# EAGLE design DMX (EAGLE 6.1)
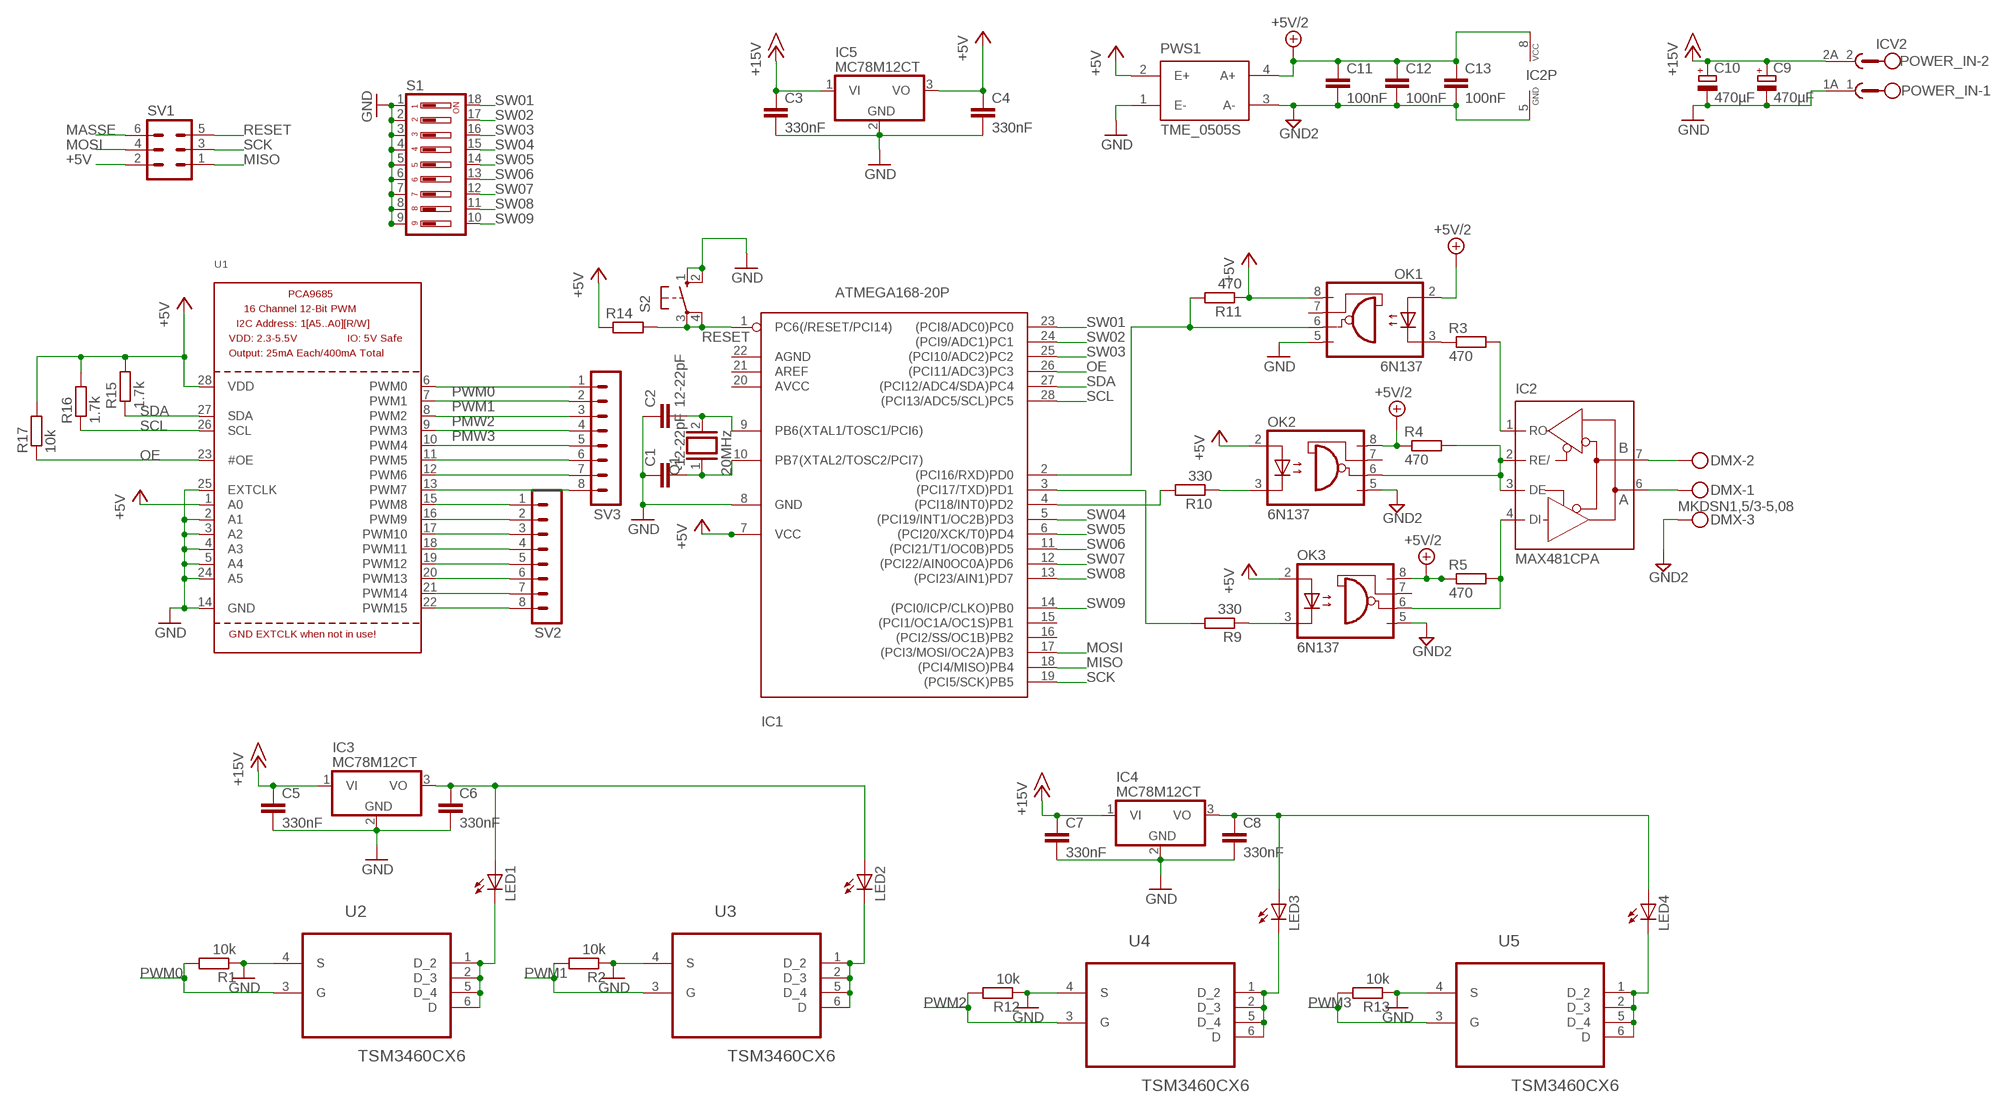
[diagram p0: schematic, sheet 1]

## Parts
C1  12-22pF  C-EU025-025X050  [C025-025X050]
C2  12-22pF  C-EU025-025X050  [C025-025X050]
C3  330nF  C-EU050-025X075  [C050-025X075]
C4  330nF  C-EU050-025X075  [C050-025X075]
C5  330nF  C-EU050-025X075  [C050-025X075]
C6  330nF  C-EU050-025X075  [C050-025X075]
C7  330nF  C-EU050-025X075  [C050-025X075]
C8  330nF  C-EU050-025X075  [C050-025X075]
C9  470µF  CPOL-EUE5-10.5  [E5-10,5]
C10  470µF  CPOL-EUE5-10.5  [E5-10,5]
C11  100nF  C-EU050-025X075  [C050-025X075]
C12  100nF  C-EU050-025X075  [C050-025X075]
C13  100nF  C-EU050-025X075  [C050-025X075]
DMX  MKDSN1,5/3-5,08  [MKDSN1,5/3-5,08]
IC1  ATMEGA168-20P  [DIL28-3]
IC2  MAX481CPA  [DIL08]
IC3  MC78M12CT  [TO220V]
IC4  MC78M12CT  [TO220V]
IC5  MC78M12CT  [TO220V]
LED1  LED5MM  [LED5MM]
LED2  LED5MM  [LED5MM]
LED3  LED5MM  [LED5MM]
LED4  LED5MM  [LED5MM]
OK1  6N137  [DIL08]
OK2  6N137  [DIL08]
OK3  6N137  [DIL08]
POWER_IN  ICV2  [ICV2]
PWS1  TME_0505S  [TMEXXXXS]
Q1  20MHz  XTAL/S  [QS]
R1  10k  R-EU_0207/7  [0207/7]
R2  10k  R-EU_0207/7  [0207/7]
R3  470  R-EU_0207/7  [0207/7]
R4  470  R-EU_0207/7  [0207/7]
R5  470  R-EU_0207/7  [0207/7]
R9  330  R-EU_0207/7  [0207/7]
R10  330  R-EU_0207/7  [0207/7]
R11  470  R-EU_0207/7  [0207/7]
R12  10k  R-EU_0207/7  [0207/7]
R13  10k  R-EU_0207/7  [0207/7]
R14  R-EU_0204/7  [0204/7]
R15  1.7k  R-EU_0204/7  [0204/7]
R16  1.7k  R-EU_0204/7  [0204/7]
R17  10k  R-EU_0204/7  [0204/7]
S1  DP09  [DP-09]
S2  10-XX  [B3F-10XX]
SV1  MA03-2  [MA03-2]
SV2  MA08-1  [MA08-1]
SV3  MA08-1  [MA08-1]
U1  PCA9685  [TSSOP28]
U2  TSM3460CX6  [SOT95P280X120-6N]
U3  TSM3460CX6  [SOT95P280X120-6N]
U4  TSM3460CX6  [SOT95P280X120-6N]
U5  TSM3460CX6  [SOT95P280X120-6N]

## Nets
+5V: C4.1 IC1.7(VCC) IC5.3(VO) OK1.8(VCC) OK2.2(A) OK3.2(A) PWS1.2(E+) R11.1 R14.1 R15.2 R16.2 R17.2 SV1.2 U1.1(A0) U1.28(VDD)
+5V/2: C11.1 C12.1 C13.1 IC2.8(VCC) OK1.2(A) OK2.8(VCC) OK3.8(VCC) PWS1.4(A+) R4.1 R5.1
+15V: C3.1 C5.1 C7.1 C9.+ C10.+ IC3.1(VI) IC4.1(VI) IC5.1(VI) POWER_IN.2A
GND: C1.1 C2.1 C3.2 C4.2 C5.2 C6.2 C7.2 C8.2 C9.- C10.- IC1.8(GND) IC3.2(GND) IC4.2(GND) IC5.2(GND) OK1.5(GND) POWER_IN.1A PWS1.1(E-) R1.1 R2.1 R12.1 R13.1 S1.1 S1.2 S1.3 S1.4 S1.5 S1.6 S1.7 S1.8 S1.9 S2.1(S) S2.2(S1) U1.2(A1) U1.3(A2) U1.4(A3) U1.5(A4) U1.14(GND) U1.24(A5) U1.25(EXTCLK) U2.4(S) U3.4(S) U4.4(S) U5.4(S)
GND2: C11.2 C12.2 C13.2 DMX.3 IC2.5(GND) OK2.5(GND) OK3.5(GND) PWS1.3(A-)
MASSE: SV1.6
MISO: IC1.18((PCI4/MISO)PB4) SV1.1
MOSI: IC1.17((PCI3/MOSI/OC2A)PB3) SV1.4
N$1: OK1.3(C) R3.1
N$2: IC2.1(RO) R3.2
N$3: IC2.2(RE/) IC2.3(DE) OK2.6(VO) R4.2
N$4: IC2.4(DI) OK3.6(VO) R5.2
N$5: OK3.3(C) R9.1
N$6: OK2.3(C) R10.1
N$7: IC1.2((PCI16/RXD)PD0) OK1.6(VO) R11.2
N$8: IC1.4((PCI18/INT0)PD2) R10.2
N$9: IC1.3((PCI17/TXD)PD1) R9.2
N$10: DMX.2 IC2.7(B)
N$11: DMX.1 IC2.6(A)
N$12: C6.1 IC3.3(VO) LED1.A LED2.A
N$13: LED3.K(C) U4.1(D_2) U4.2(D_3) U4.5(D_4) U4.6(D)
N$14: C8.1 IC4.3(VO) LED3.A LED4.A
N$15: LED1.K(C) U2.1(D_2) U2.2(D_3) U2.5(D_4) U2.6(D)
N$16: LED4.K(C) U5.1(D_2) U5.2(D_3) U5.5(D_4) U5.6(D)
N$17: LED2.K(C) U3.1(D_2) U3.2(D_3) U3.5(D_4) U3.6(D)
N$18: C1.2 IC1.10(PB7(XTAL2/TOSC2/PCI7)) Q1.1
N$19: C2.2 IC1.9(PB6(XTAL1/TOSC1/PCI6)) Q1.2
N$22: SV3.5 U1.10(PWM4)
N$23: SV3.6 U1.11(PWM5)
N$24: SV3.7 U1.12(PWM6)
N$25: SV3.8 U1.13(PWM7)
N$26: SV2.1 U1.15(PWM8)
N$27: SV2.2 U1.16(PWM9)
N$28: SV2.3 U1.17(PWM10)
N$29: SV2.4 U1.18(PWM11)
N$30: SV2.5 U1.19(PWM12)
N$31: SV2.6 U1.20(PWM13)
N$32: SV2.7 U1.21(PWM14)
N$33: SV2.8 U1.22(PWM15)
OE: IC1.26((PCI11/ADC3)PC3) R17.1 U1.23(#OE)
PMW2: SV3.3 U1.8(PWM2)
PMW3: SV3.4 U1.9(PWM3)
PWM0: R1.2 SV3.1 U1.6(PWM0) U2.3(G)
PWM1: R2.2 SV3.2 U1.7(PWM1) U3.3(G)
PWM2: R12.2 U4.3(G)
PWM3: R13.2 U5.3(G)
RESET: IC1.1(PC6(/RESET/PCI14)) R14.2 S2.3(P) S2.4(P1) SV1.5
SCK: IC1.19((PCI5/SCK)PB5) SV1.3
SCL: IC1.28((PCI13/ADC5/SCL)PC5) R16.1 U1.26(SCL)
SDA: IC1.27((PCI12/ADC4/SDA)PC4) R15.1 U1.27(SDA)
SW01: IC1.23((PCI8/ADC0)PC0) S1.18
SW02: IC1.24((PCI9/ADC1)PC1) S1.17
SW03: IC1.25((PCI10/ADC2)PC2) S1.16
SW04: IC1.5((PCI19/INT1/OC2B)PD3) S1.15
SW05: IC1.6((PCI20/XCK/T0)PD4) S1.14
SW06: IC1.11((PCI21/T1/OC0B)PD5) S1.13
SW07: IC1.12((PCI22/AIN0OC0A)PD6) S1.12
SW08: IC1.13((PCI23/AIN1)PD7) S1.11
SW09: IC1.14((PCI0/ICP/CLKO)PB0) S1.10
Unconnected: IC1.15((PCI1/OC1A/OC1S)PB1) IC1.16((PCI2/SS/OC1B)PB2) IC1.20(AVCC) IC1.21(AREF) IC1.22(AGND) OK1.7(VE) OK2.7(VE) OK3.7(VE) POWER_IN.1 POWER_IN.2

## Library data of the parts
C1-C8 C11-C13 = rcl:C-EU: CAPACITOR, European symbol
C9 C10 = rcl:CPOL-EU: POLARIZED CAPACITOR, European symbol
DMX = con-phoenix-508:MKDSN1,5/3-5,08: MKDSN 1,5/ 3-5,08 Printklemme Nennstrom: 13,5 A Nennspannung: 250 V Rastermaß: 5,08 mm Polzahl: 3 Anschlussart: Schraubanschluss Montage: Löten Anschlussrichtung Leiter/Platine: 0 ° Artikelnummer: 1729131 Source: http://eshop.phoenixcontact.com .. 1729131.pdf; MPN: SMKDSN1,5/3-5,08; OC_FARNELL: 1792904; OC_NEWARK: 70R0299
IC1 = adafruit:ATMEGA168*P: MICROCONTROLLER 16 kBytes FLASH 1 kBytes SRAM 512 Bytes EEPROM USART 8-channel 10 bit ADC
IC2 = maxim:MAX481CPA: RS485 TRANSEIVER; MPN: MAX485; OC_FARNELL: unknown; OC_NEWARK: 99K3445
IC3-IC5 = linear:MC78M: 500 mA Positive Voltage Regulators Source: Data sheet
LED1-LED4 = led:LED: LED
OK1-OK3 = optocoupler:6N137: MOTOROLA OPTO COUPLER; MPN: 6N137; OC_FARNELL: 1328376; OC_NEWARK: 52M1895
POWER_IN = con-phoenix-508:ICV2: PHOENIX; OC_FARNELL: unknown; OC_NEWARK: unknown
PWS1 = traco-electronic:TME_*S: DC/DC Konverter 1 Watt Source: http://www.tracopower.com/datasheet_g/tme-d.pdf; MPN: TME 0505S; OC_FARNELL: 1007538; OC_NEWARK: 51R5321
Q1 = special:XTAL/S: CRYSTAL
R1-R5 R9-R17 = rcl:R-EU_: RESISTOR, European symbol
S1 = switch-dil:DP09: DIL/CODE SWITCH; MPN: MCDP09; OC_FARNELL: 1522007; OC_NEWARK: 74M2979
S2 = switch-omron:10-XX: OMRON SWITCH; MPN: B3F-1000; OC_FARNELL: 176432; OC_NEWARK: 36M3542
SV1 = con-lstb:MA03-2: PIN HEADER; OC_FARNELL: unknown; OC_NEWARK: unknown
SV2 SV3 = con-lstb:MA08-1: PIN HEADER; OC_FARNELL: unknown; OC_NEWARK: unknown
U1 = adafruit:PCA9685: PCA9685 - 16 Channel 12-Bit I2C PWM Controller 5.0V tolerant 16 channel, 12-bit I2C PWM controller with 25mA per output (max. 400mA total) Digikey: 568-5931-1-ND
U2-U5 = farnell:TSM3460CX6: N-Channel MOSFET; MPN: TSM3460CX6; OC_FARNELL: 1864595; OC_NEWARK: 27T3007; PACKAGE: SOT-6; SUPPLIER: Taiwan Semiconductors

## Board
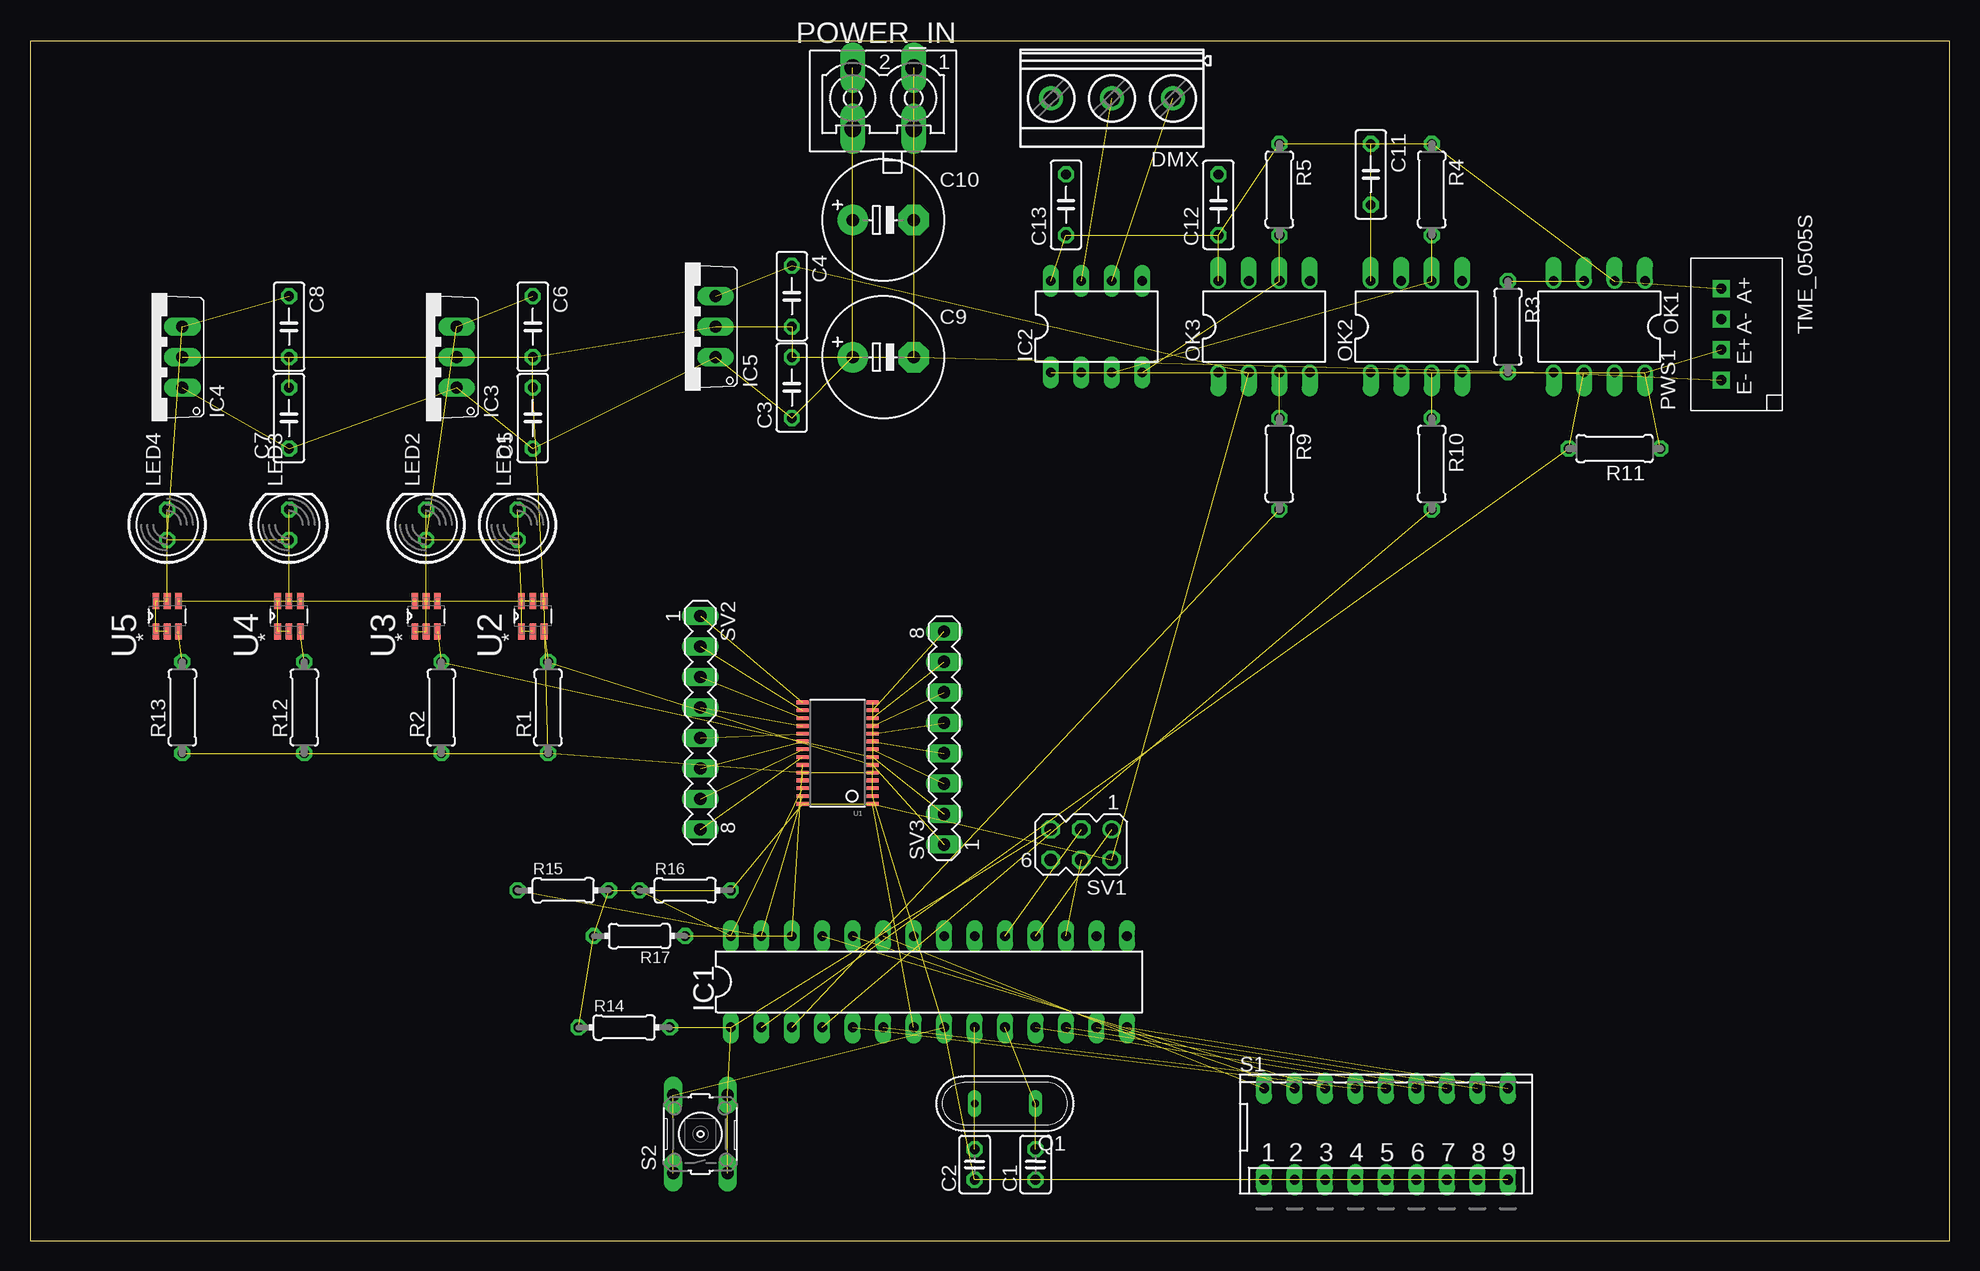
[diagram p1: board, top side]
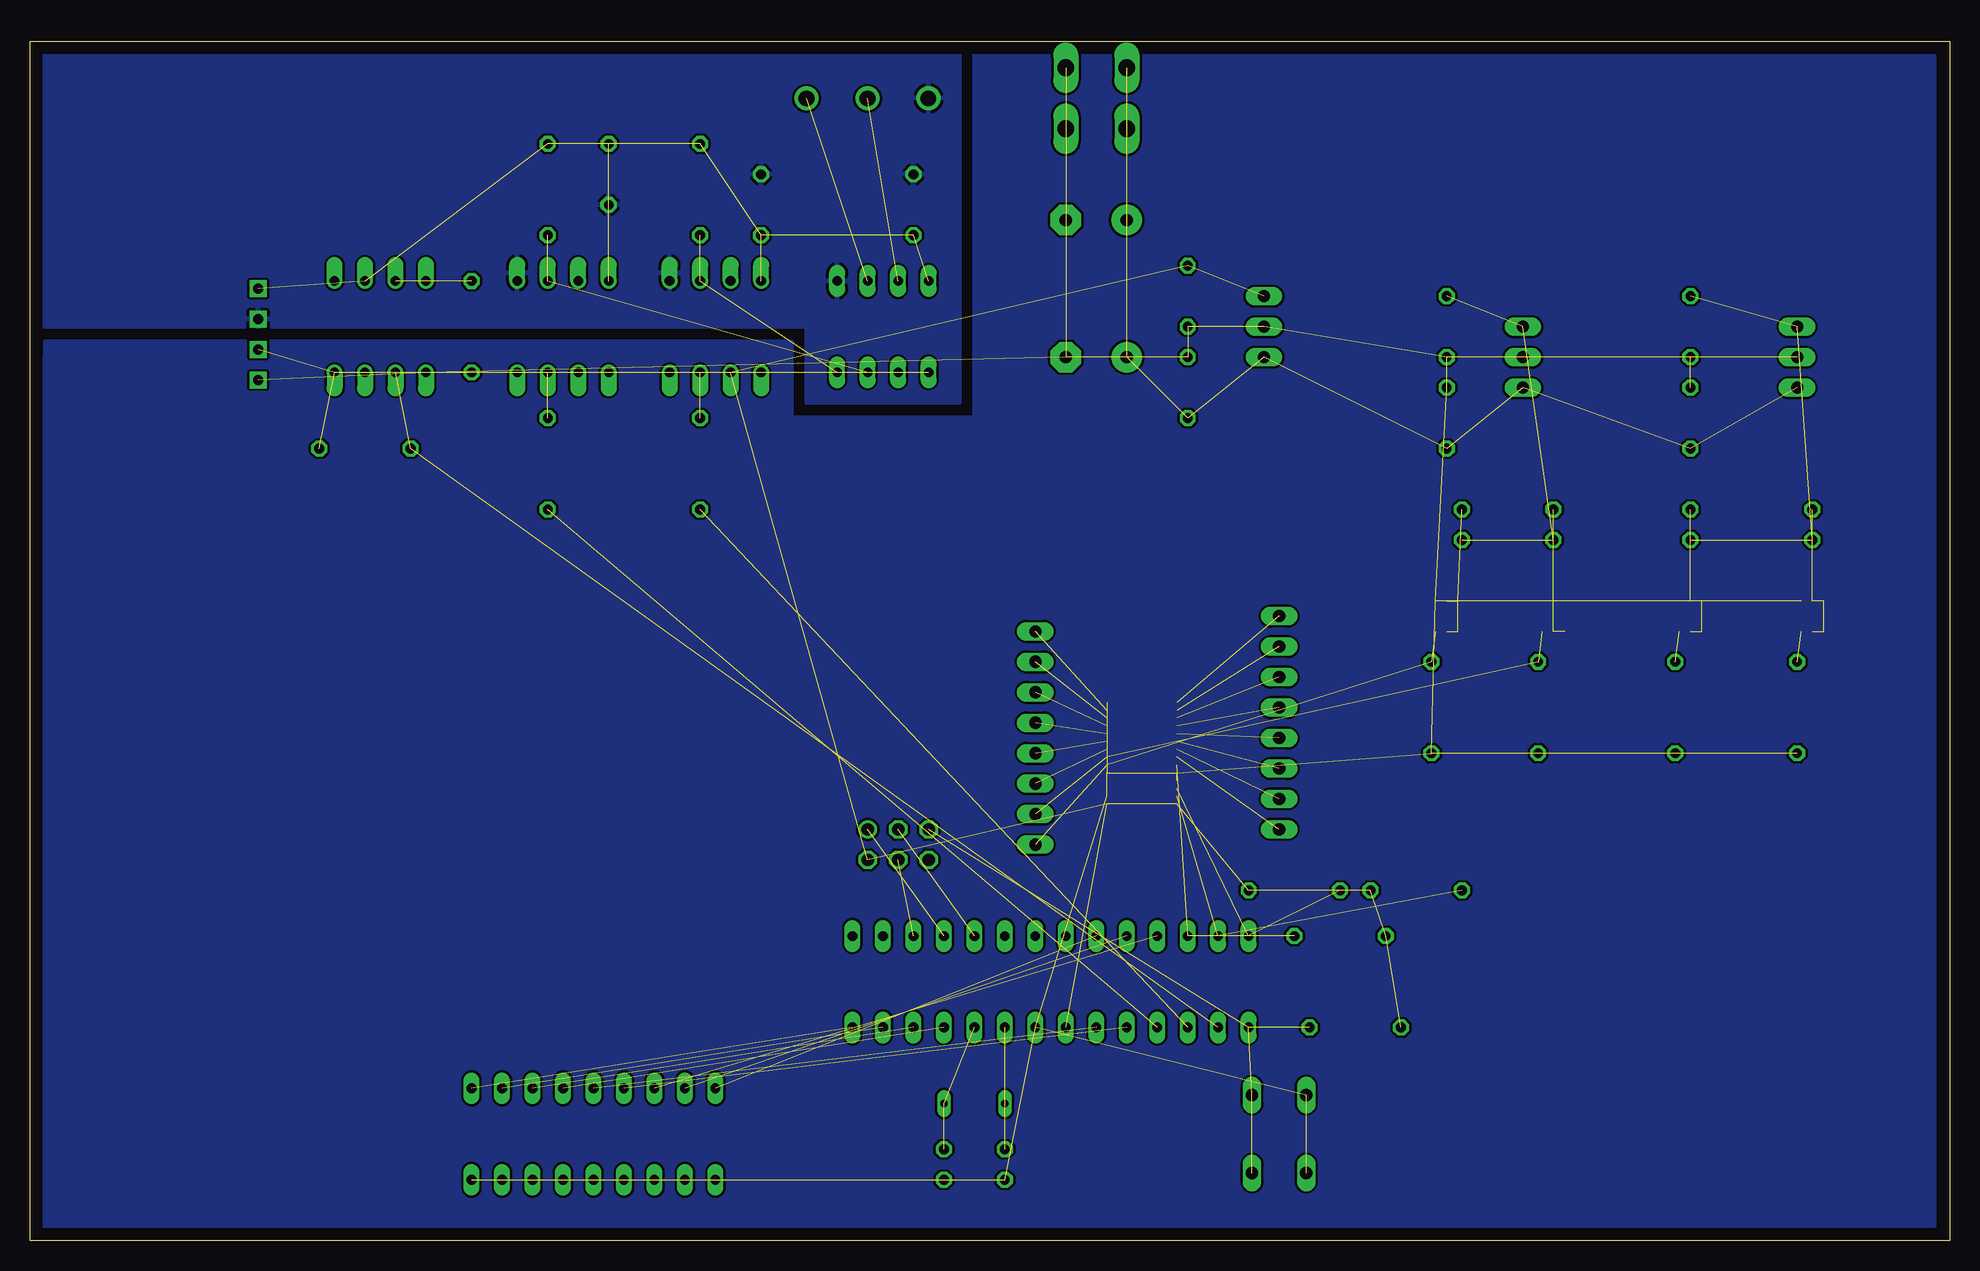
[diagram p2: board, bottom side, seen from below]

Size 160 x 100 mm. Coordinates in mm from the lower left corner, seen from the top.
Outline: 0,0 160,0 160,100 0,100 0,0
Copper layers (1*16): Top 0.035mm / dielectric 1.5mm / Bottom 0.035mm
Design rules: minimum track width 10mil, minimum drill 24mil, track to track 8mil, track to pad 8mil, pad to pad 8mil, via to via 8mil, smd to smd 8mil, copper to edge 40mil, drill to drill 8mil, minimum pad ring 10mil, minimum via ring 8mil, stop-mask expansion 4mil, vias tented up to drill 0mil, thermal gap 10mil

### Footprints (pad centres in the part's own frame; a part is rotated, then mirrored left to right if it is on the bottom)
C025-025X050 = drill 0.813 octagon: 1 -1.27,0; 2 1.27,0
C050-025X075 = drill 0.813 octagon: 1 -2.54,0; 2 2.54,0
E5-10,5 = drill 1.016 pad 2.54: + -2.54,0 | drill 1.016 pad 2.54 octagon: - 2.54,0
MKDSN1,5/3-5,08 = drill 1.3 pad 2: 1 -7.641,0.025; 2 -2.561,0.025; 3 2.519,0.025
DIL28-3 = drill 0.813 long: 1 -16.51,-3.81; 2 -13.97,-3.81; 3 -11.43,-3.81; 4 -8.89,-3.81; 5 -6.35,-3.81; 6 -3.81,-3.81; 7 -1.27,-3.81; 8 1.27,-3.81; 9 3.81,-3.81; 10 6.35,-3.81; 11 8.89,-3.81; 12 11.43,-3.81; 13 13.97,-3.81; 14 16.51,-3.81; 15 16.51,3.81; 16 13.97,3.81; 17 11.43,3.81; 18 8.89,3.81; 19 6.35,3.81; 20 3.81,3.81; 21 1.27,3.81; 22 -1.27,3.81; 23 -3.81,3.81; 24 -6.35,3.81; 25 -8.89,3.81; 26 -11.43,3.81; 27 -13.97,3.81; 28 -16.51,3.81
DIL08 = drill 0.813 long: 1 -3.81,-3.81; 2 -1.27,-3.81; 3 1.27,-3.81; 4 3.81,-3.81; 5 3.81,3.81; 6 1.27,3.81; 7 -1.27,3.81; 8 -3.81,3.81
TO220V = drill 1.016 long: 1 -2.54,-2.54; 2 0,-2.54; 3 2.54,-2.54
LED5MM = drill 0.813 octagon: A -1.27,0; K 1.27,0
DIL08' = drill 0.813 offset: 1 -3.81,-3.81; 2 -1.27,-3.81; 3 1.27,-3.81; 4 3.81,-3.81; 5 3.81,3.81; 6 1.27,3.81; 7 -1.27,3.81; 8 -3.81,3.81
ICV2 = drill 1.397 long: 1 -2.54,2.54; 1A -2.54,-2.54; 2 2.54,2.54; 2A 2.54,-2.54
TMEXXXXS = drill 0.813 pad 1.397 square: 1 -3.81,1.27; 2 -1.27,1.27; 3 1.27,1.27; 4 3.81,1.27
QS = drill 0.61 long: 1 -2.54,0; 2 2.54,0
0207/7 = drill 0.813 octagon: 1 -3.81,0; 2 3.81,0
0204/7 = drill 0.813 octagon: 1 -3.81,0; 2 3.81,0
DP-09 = drill 0.813 long: 1 -10.16,-3.81; 2 -7.62,-3.81; 3 -5.08,-3.81; 4 -2.54,-3.81; 5 0,-3.81; 6 2.54,-3.81; 7 5.08,-3.81; 8 7.62,-3.81; 9 10.16,-3.81; 10 10.16,3.81; 11 7.62,3.81; 12 5.08,3.81; 13 2.54,3.81; 14 0,3.81; 15 -2.54,3.81; 16 -5.08,3.81; 17 -7.62,3.81; 18 -10.16,3.81
B3F-10XX = drill 1.016 long: 1 -3.251,2.261; 2 3.251,2.261; 3 -3.251,-2.261; 4 3.251,-2.261
MA03-2 = drill 1.016: 1 -2.54,-1.27 | drill 1.016 octagon: 2 -2.54,1.27; 3 0,-1.27; 4 0,1.27; 5 2.54,-1.27; 6 2.54,1.27
MA08-1 = drill 1.016 long: 1 -8.89,0; 2 -6.35,0; 3 -3.81,0; 4 -1.27,0; 5 1.27,0; 6 3.81,0; 7 6.35,0; 8 8.89,0
TSSOP28 = smd 0.305 x 0.991: 1 -4.225,-2.918; 2 -3.575,-2.918; 3 -2.925,-2.918; 4 -2.275,-2.918; 5 -1.625,-2.918; 6 -0.975,-2.918; 7 -0.325,-2.918; 8 0.325,-2.918; 9 0.975,-2.918; 10 1.625,-2.918; 11 2.275,-2.918; 12 2.925,-2.918; 13 3.575,-2.918; 14 4.225,-2.918; 15 4.225,2.918; 16 3.575,2.918; 17 2.925,2.918; 18 2.275,2.918; 19 1.625,2.918; 20 0.975,2.918; 21 0.325,2.918; 22 -0.325,2.918; 23 -0.975,2.918; 24 -1.625,2.918; 25 -2.275,2.918; 26 -2.925,2.918; 27 -3.575,2.918; 28 -4.225,2.918
SOT95P280X120-6N = smd 1.321 x 0.559: 1 -1.27,0.94; 2 -1.27,0; 3 -1.27,-0.94; 4 1.27,-0.94; 5 1.27,0; 6 1.27,0.94

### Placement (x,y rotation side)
C1  83.82,6.35 90 top
C2  78.74,6.35 90 top
C3  63.5,71.12 90 top
C4  63.5,78.74 270 top
C5  41.91,68.58 90 top
C6  41.91,76.2 270 top
C7  21.59,68.58 90 top
C8  21.59,76.2 270 top
C9  71.12,73.66 0 top
C10  71.12,85.09 0 top
C11  111.76,88.9 270 top
C12  99.06,86.36 90 top
C13  86.36,86.36 90 top
DMX  87.63,95.25 180 top
IC1  74.93,21.59 0 top
IC2  88.9,76.2 0 top
IC3  33.02,73.66 90 top
IC4  10.16,73.66 90 top
IC5  54.61,76.2 90 top
LED1  40.64,59.69 90 top
LED2  33.02,59.69 90 top
LED3  21.59,59.69 90 top
LED4  11.43,59.69 90 top
OK1  6N137  [DIL08']  130.81,76.2 180 top
OK2  6N137  [DIL08']  115.57,76.2 0 top
OK3  6N137  [DIL08']  102.87,76.2 0 top
POWER_IN  71.12,95.25 180 top
PWS1  142.24,75.56 90 top
Q1  81.28,11.43 180 top
R1  43.18,44.45 90 top
R2  34.29,44.45 90 top
R3  123.19,76.2 270 top
R4  116.84,87.63 270 top
R5  104.14,87.63 270 top
R9  104.14,64.77 270 top
R10  116.84,64.77 270 top
R11  132.08,66.04 180 top
R12  22.86,44.45 90 top
R13  12.7,44.45 90 top
R14  49.53,17.78 0 top
R15  44.45,29.21 0 top
R16  54.61,29.21 0 top
R17  50.8,25.4 180 top
S1  113.03,8.89 0 top
S2  55.88,8.89 90 top
SV1  87.63,33.02 180 top
SV2  55.88,43.18 270 top
SV3  76.2,41.91 90 top
U1  67.31,40.64 90 top
U2  41.91,52.07 90 top
U3  33.02,52.07 90 top
U4  21.59,52.07 90 top
U5  11.43,52.07 90 top

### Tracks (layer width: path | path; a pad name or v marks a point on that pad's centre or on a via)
+5V  (14 unrouted)
+5V/2  (9 unrouted)
+15V  (8 unrouted)
GND  (42 unrouted)
GND2
  pour Bottom: 82.55,99.06 82.55,69.85 95.25,69.85 95.25,76.2 158.75,76.2 158.75,99.06
MISO  (1 unrouted)
MOSI  (1 unrouted)
N$1  (1 unrouted)
N$2  (1 unrouted)
N$3  (3 unrouted)
N$4  (2 unrouted)
N$5  (1 unrouted)
N$6  (1 unrouted)
N$7  (2 unrouted)
N$8  (1 unrouted)
N$9  (1 unrouted)
N$10  (1 unrouted)
N$11  (1 unrouted)
N$12  (3 unrouted)
N$13  (4 unrouted)
N$14  (3 unrouted)
N$15  (4 unrouted)
N$16  (4 unrouted)
N$17  (4 unrouted)
N$18  (2 unrouted)
N$19  (2 unrouted)
N$20
  pour Bottom: 1.27,99.06 81.28,99.06 81.28,68.58 96.52,68.58 96.52,74.93 158.75,74.93 160.02,1.27 1.27,1.27
N$22  (1 unrouted)
N$23  (1 unrouted)
N$24  (1 unrouted)
N$25  (1 unrouted)
N$26  (1 unrouted)
N$27  (1 unrouted)
N$28  (1 unrouted)
N$29  (1 unrouted)
N$30  (1 unrouted)
N$31  (1 unrouted)
N$32  (1 unrouted)
N$33  (1 unrouted)
OE  (2 unrouted)
PMW2  (1 unrouted)
PMW3  (1 unrouted)
PWM0  (3 unrouted)
PWM1  (3 unrouted)
PWM2  (1 unrouted)
PWM3  (1 unrouted)
RESET  (4 unrouted)
SCK  (1 unrouted)
SCL  (2 unrouted)
SDA  (2 unrouted)
SW01  (1 unrouted)
SW02  (1 unrouted)
SW03  (1 unrouted)
SW04  (1 unrouted)
SW05  (1 unrouted)
SW06  (1 unrouted)
SW07  (1 unrouted)
SW08  (1 unrouted)
SW09  (1 unrouted)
